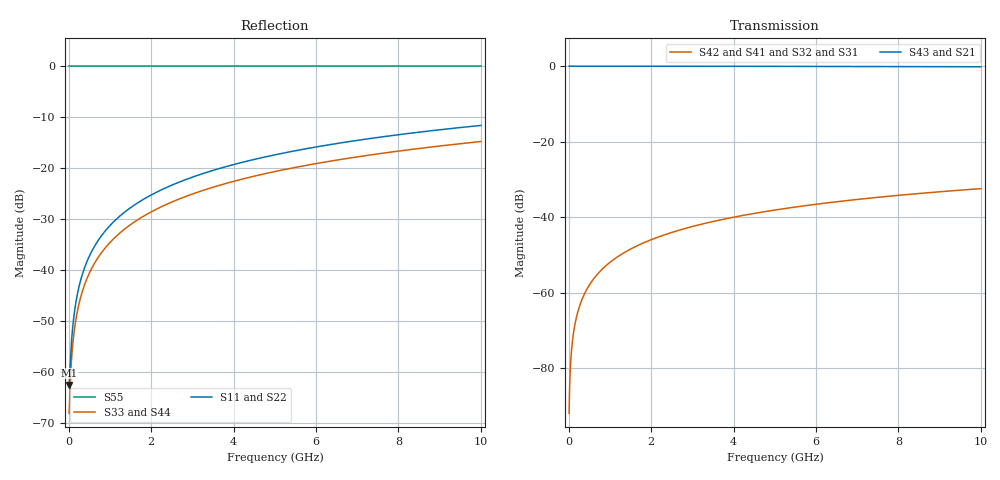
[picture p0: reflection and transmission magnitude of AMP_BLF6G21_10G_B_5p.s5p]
! Created Wed Feb 17 11:28:34 2010
# ghz S ma R 50
! 5 Port Network Data from SP1.SP block
! freq  magS11  angS11  magS12  angS12  magS13  angS13  magS14  angS14
!  magS15  angS15
!  magS21  angS21  magS22  angS22  magS23  angS23
!  magS24  angS24  magS25  angS25
!  magS31  angS31  magS32  angS32
!  magS33  angS33  magS34  angS34  magS35  angS35
!  magS41  angS41
!  magS42  angS42  magS43  angS43  magS44  angS44  magS45  angS45
!  magS51  angS51  magS52  angS52  magS53  angS53  magS54  angS54
!  magS55  angS55
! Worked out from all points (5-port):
!   1000 points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, 10 MHz to 10 GHz, reference 50 ohm
!   strongest paths, dB at 10 MHz, 2.51 GHz, 5.01 GHz, 7.51 GHz, 10 GHz:
!     S43: 0.0, 0.0, 0.0, -0.1, -0.2
!     S21: 0.0, 0.0, -0.1, -0.2, -0.3
!     S42: -91.9, -44.0, -38.1, -34.7, -32.4
!     S41: -91.9, -44.0, -38.1, -34.7, -32.4
!     S32: -91.9, -44.0, -38.1, -34.7, -32.4
!     S31: -91.9, -44.0, -38.1, -34.7, -32.4
!   lowest |S11| = -62.6 dB at 10 MHz (marker M1), VSWR 1.00, Z = 50.1 + j0.0273 ohm
!   |S11| at or under -10 dB: start of sweep to end of sweep
